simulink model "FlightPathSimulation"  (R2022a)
settings: Solver=VariableStepAuto  StartTime=0.0  StopTime=TF  RelTol=1e-3
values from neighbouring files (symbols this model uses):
  aircraft = RCAM_Transport    [RunSimulation.m]
undefined symbols (not defined in the file or in its folder): Column, Controls_0, D, deg, Earth, ft, km, m, rad, s, States_0, vector, WGS84
libraries: aerolibconvert2 x19, aerolibasang x3, aerolibadyn x1, aerolibatmos2 x1, shared6dof x1, aerolibtransform2 x1

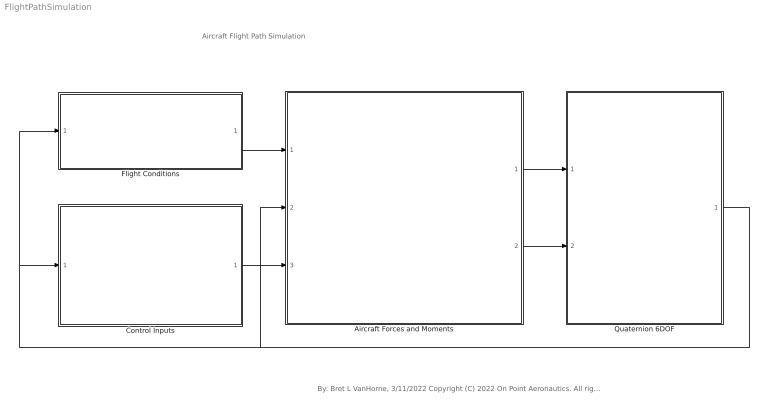
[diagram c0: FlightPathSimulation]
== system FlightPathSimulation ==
  note: Aircraft Flight Path Simulation
  note: By: Bret L VanHorne, 3/11/2022 Copyright (C) 2022 On Point Aeronautics. All rights reserved.
  Aircraft Forces and Moments : Subsystem
  Control Inputs : Subsystem
  Flight Conditions : Subsystem
  Quaternion 6DOF : Subsystem
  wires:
  Quaternion 6DOF/1(Bus Element Out13) -> Flight Conditions/1(Bus Element In2), Control Inputs/1(Bus Element In4), Aircraft Forces and Moments/3(States)
  Flight Conditions/1(Bus Element Out6) -> Aircraft Forces and Moments/1(Conditions)
  Control Inputs/1(Bus Element Out1) -> Aircraft Forces and Moments/2(Controls)
  Aircraft Forces and Moments/1(Forces) -> Quaternion 6DOF/1(Forces)
  Aircraft Forces and Moments/2(Moments) -> Quaternion 6DOF/2(Moments)

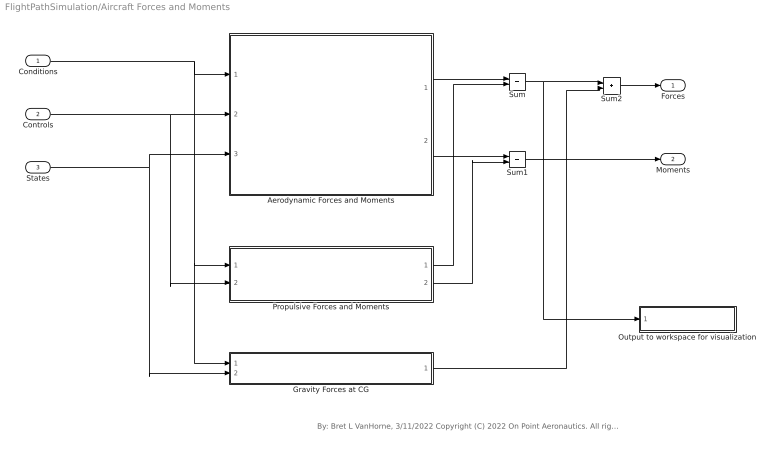
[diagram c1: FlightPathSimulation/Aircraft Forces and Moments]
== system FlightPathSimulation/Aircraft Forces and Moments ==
  note: By: Bret L VanHorne, 3/11/2022 Copyright (C) 2022 On Point Aeronautics. All rights reserved.
  Conditions : Inport
  Controls : Inport  Port=2
  States : Inport  Port=3
  Aerodynamic Forces and Moments : Subsystem
  Gravity Forces at CG : Subsystem
  Output to workspace for visualization : Subsystem
  Propulsive Forces and Moments : Subsystem
  Sum : Sum
  Sum1 : Sum
  Sum2 : Sum
  Forces : Outport
  Moments : Outport  Port=2
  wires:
  Aerodynamic Forces and Moments/1(Forces) -> Sum/1
  Propulsive Forces and Moments/1(Forces) -> Sum/2
  Aerodynamic Forces and Moments/2(Moments) -> Sum1/1
  Propulsive Forces and Moments/2(Moments) -> Sum1/2
  Conditions/1 -> Gravity Forces at CG/1(Bus Element In1), Propulsive Forces and Moments/1(Bus Element In), Aerodynamic Forces and Moments/1(Bus Element In9)
  Sum1/1 -> Moments/1
  Controls/1 -> Aerodynamic Forces and Moments/2(Bus Element In14), Propulsive Forces and Moments/2(Bus Element In2)
  States/1 -> Aerodynamic Forces and Moments/3(Bus Element In11), Gravity Forces at CG/2(Bus Element In2)
  Sum/1 -> Sum2/1, Output to workspace for visualization/1(In1)
  Gravity Forces at CG/1(Forces) -> Sum2/2
  Sum2/1 -> Forces/1

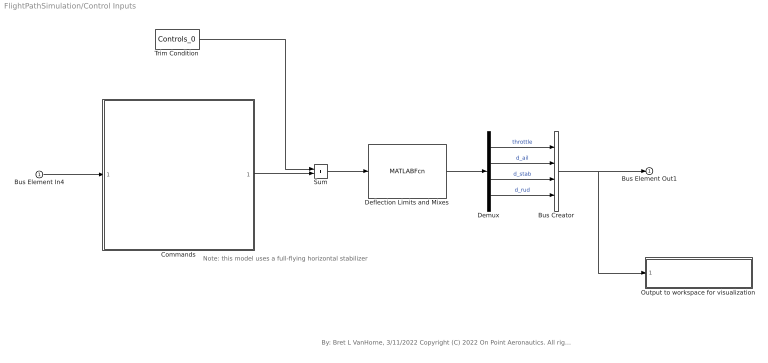
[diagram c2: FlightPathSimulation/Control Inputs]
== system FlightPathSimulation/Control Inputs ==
  note: Note: this model uses a full-flying horizontal stabilizer
  note: By: Bret L VanHorne, 3/11/2022 Copyright (C) 2022 On Point Aeronautics. All rights reserved.
  Bus Element In4 : Inport
  Bus Creator : BusCreator  Inputs=4
  Commands : Subsystem  ReferencedSubsystem=TurnCommands
  Deflection Limits and Mixes : MATLABFcn  MATLABFcn=aircraft.ControlRigging(u)
  Demux : Demux
  Output to workspace for visualization : Subsystem
  Sum : Sum
  Trim Condition : Constant  Value=Controls_0
  Bus Element Out1 : Outport
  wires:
  Sum/1 -> Deflection Limits and Mixes/1
  Trim Condition/1 -> Sum/1
  Bus Creator/1 -> Output to workspace for visualization/1(In1), Bus Element Out1/1
  Bus Element In4/1 -> Commands/1
  Commands/1 -> Sum/2
  Deflection Limits and Mixes/1 -> Demux/1
  Demux/1 -> Bus Creator/1  "throttle"
  Demux/2 -> Bus Creator/2  "d_ail"
  Demux/3 -> Bus Creator/3  "d_stab"
  Demux/4 -> Bus Creator/4  "d_rud"

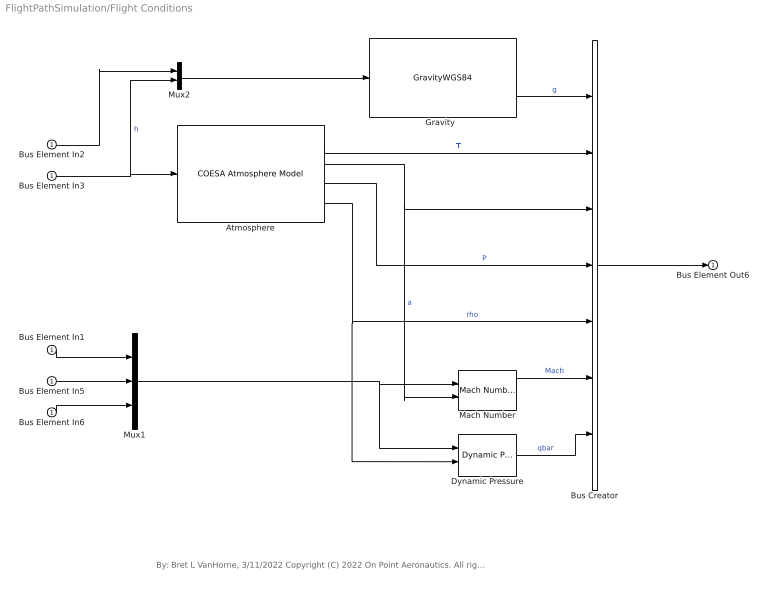
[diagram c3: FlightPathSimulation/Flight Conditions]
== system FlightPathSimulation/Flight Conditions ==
  note: By: Bret L VanHorne, 3/11/2022 Copyright (C) 2022 On Point Aeronautics. All rights reserved.
  Bus Element In{1..3,5..6} (5 alike) : Inport
  Atmosphere : aerolibatmos2/COESA Atmosphere Model  units=Metric (MKS)  spec=1976 COESA-extended U.S. Standard Atmosphere  model=Profile  profile_var=High temperature  profile_percent=1%  profile_alt=5 km (16404 ft)  envelope_var=High temperature  envelope_percent=1%  action=Warning
  Bus Creator : BusCreator  Inputs=7
  Dynamic Pressure : aerolibasang/Dynamic Pressure
  "Gravity  " : GravityWGS84
  Mach Number : aerolibasang/Mach Number
  Mux1 : Mux  Inputs=3
  Mux2 : Mux  Inputs=2
  Bus Element Out6 : Outport
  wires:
  Bus Element In6/1 -> Mux1/3
  Bus Element In5/1 -> Mux1/2
  Bus Element In2/1 -> Mux2/1
  Bus Element In1/1 -> Mux1/1
  Dynamic Pressure/1 -> Bus Creator/7  "qbar"
  Atmosphere/3 -> Bus Creator/4  "P"
  Atmosphere/1 -> Bus Creator/2  "T"
  Mux2/1 -> "Gravity  "/1
  Atmosphere/4 -> Dynamic Pressure/2, Bus Creator/5  "rho"
  "Gravity  "/1 -> Bus Creator/1  "g"
  Atmosphere/2 -> Mach Number/2, Bus Creator/3  "a"
  Mach Number/1 -> Bus Creator/6  "Mach"
  Bus Element In3/1 -> Mux2/2, Atmosphere/1  "h"
  Mux1/1 -> Dynamic Pressure/1, Mach Number/1
  Bus Creator/1 -> Bus Element Out6/1

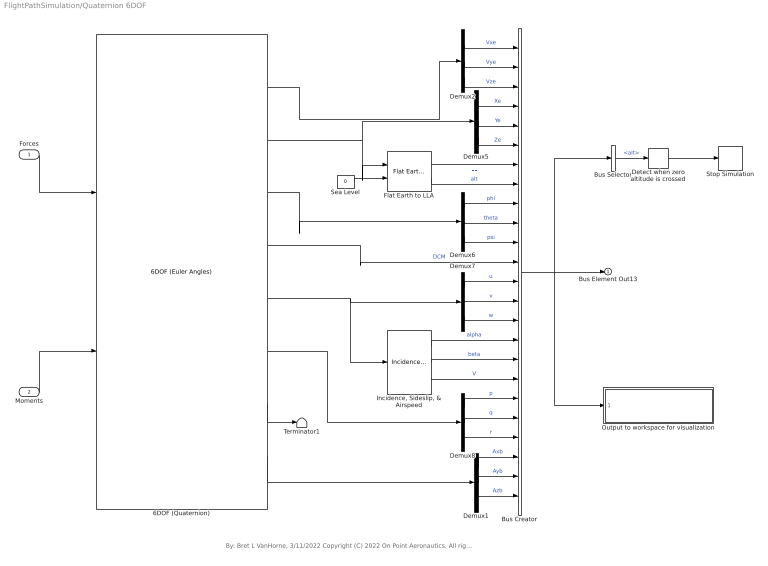
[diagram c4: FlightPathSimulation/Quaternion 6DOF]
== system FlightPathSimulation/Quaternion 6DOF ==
  note: By: Bret L VanHorne, 3/11/2022 Copyright (C) 2022 On Point Aeronautics. All rights reserved.
  Forces : Inport
  Moments : Inport  Port=2
  6DOF (Quaternion) : shared6dof/6DOF (Euler Angles)  units=Metric (MKS)  mtype=Fixed  rep=Quaternion  xme_0=States_0(1,:)  Vm_0=States_0(2,:)  eul_0=Euler_0  pm_0=States_0(3,:)  mass_0=aircraft.mass  mass_e=0.5  mass_f=2.0  inertia=aircraft.I  inertia_e=eye(3)  inertia_f=2*eye(3)  k_quat=1.0  vre_flag=on  abi_flag=off  aMode=0  xme_statename=''  Vm_statename=''  eul_statename=''  quat_statename=''  pm_statename=''  mass_statename=''
  Bus Selector : BusSelector  OutputSignals=alt
  Bus Creator : BusCreator  Inputs=24
  Demux{1..2,5..8} (6 alike) : Demux  Outputs=3
  Detect when zero altitude is crossed : HitCross
  Flat Earth to LLA : aerolibtransform2/Flat Earth to LLA  units=Metric (MKS)  ptype=Earth (WGS84)  F=1/298.257223563  R=6378137  refPosPort=off  LL0=[0 10]  psi=0
  "Incidence, Sideslip, & Airspeed" : aerolibasang/Incidence, Sideslip, & Airspeed
  Output to workspace for visualization : Subsystem
  Sea Level : Constant  Value=0
  Stop Simulation : Stop
  Terminator1 : Terminator
  Bus Element Out13 : Outport
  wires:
  Moments/1 -> 6DOF (Quaternion)/2
  Forces/1 -> 6DOF (Quaternion)/1
  6DOF (Quaternion)/2 -> Flat Earth to LLA/1, Demux5/1
  6DOF (Quaternion)/3 -> Demux6/1
  6DOF (Quaternion)/5 -> Demux7/1, "Incidence, Sideslip, & Airspeed"/1
  6DOF (Quaternion)/6 -> Demux8/1
  6DOF (Quaternion)/7 -> Terminator1/1
  6DOF (Quaternion)/1 -> Demux2/1
  Demux5/1 -> Bus Creator/4  "Xe"
  Demux5/2 -> Bus Creator/5  "Ye"
  Demux5/3 -> Bus Creator/6  "Ze"
  Demux6/1 -> Bus Creator/9  "phi"
  Demux6/2 -> Bus Creator/10  "theta"
  Demux6/3 -> Bus Creator/11  "psi"
  Demux7/1 -> Bus Creator/13  "u"
  Demux7/2 -> Bus Creator/14  "v"
  Demux7/3 -> Bus Creator/15  "w"
  Demux8/1 -> Bus Creator/19  "p"
  Demux8/2 -> Bus Creator/20  "q"
  Demux8/3 -> Bus Creator/21  "r"
  6DOF (Quaternion)/4 -> Bus Creator/12  "DCM"
  Bus Creator/1 -> Output to workspace for visualization/1(In1), Bus Element Out13/1, Bus Selector/1
  6DOF (Quaternion)/8 -> Demux1/1
  Demux1/1 -> Bus Creator/22  "Axb"
  Demux1/2 -> Bus Creator/23  "Ayb"
  Demux1/3 -> Bus Creator/24  "Azb"
  Bus Selector/1 -> Detect when zero altitude is crossed/1  "<alt>"
  Detect when zero altitude is crossed/1 -> Stop Simulation/1
  Demux2/1 -> Bus Creator/1  "Vxe"
  Demux2/2 -> Bus Creator/2  "Vye"
  Demux2/3 -> Bus Creator/3  "Vze"
  "Incidence, Sideslip, & Airspeed"/1 -> Bus Creator/16  "alpha"
  "Incidence, Sideslip, & Airspeed"/2 -> Bus Creator/17  "beta"
  "Incidence, Sideslip, & Airspeed"/3 -> Bus Creator/18  "V"
  Sea Level/1 -> Flat Earth to LLA/2
  Flat Earth to LLA/1 -> Bus Creator/7  "LL"
  Flat Earth to LLA/2 -> Bus Creator/8  "alt"

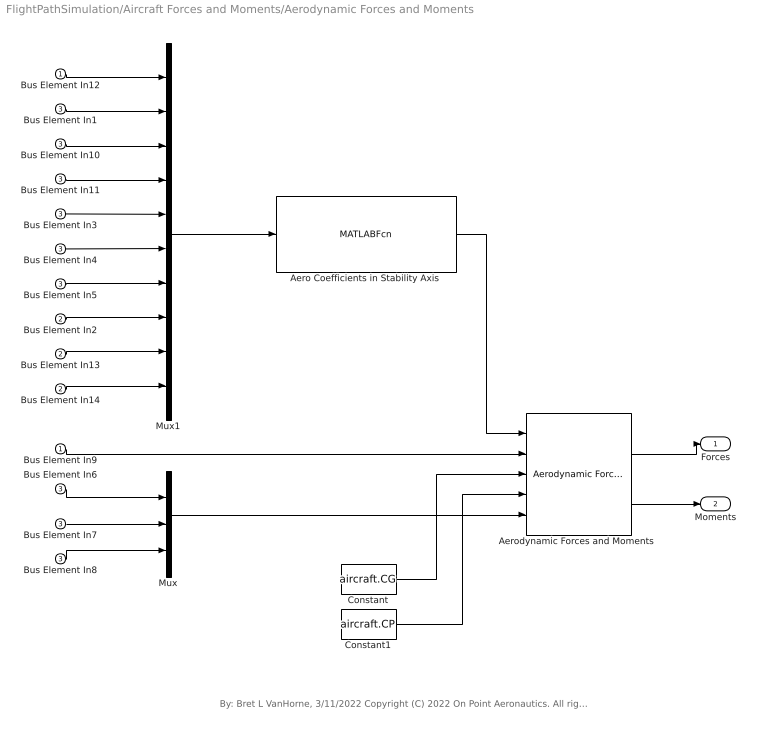
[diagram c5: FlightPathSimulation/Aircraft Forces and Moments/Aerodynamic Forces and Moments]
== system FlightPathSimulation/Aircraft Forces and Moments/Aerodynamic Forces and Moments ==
  note: By: Bret L VanHorne, 3/11/2022 Copyright (C) 2022 On Point Aeronautics. All rights reserved.
  Bus Element In9 : Inport
  Bus Element In12 : Inport
  Bus Element In2 : Inport  Port=2
  Bus Element In13 : Inport  Port=2
  Bus Element In14 : Inport  Port=2
  Bus Element In{1,3..8,10..11} (9 alike) : Inport  Port=3
  Aero Coefficients in Stability Axis : MATLABFcn  MATLABFcn=aircraft.AeroCoefficients(u(1), u(2:7), u(8:10))
  "Aerodynamic Forces and Moments " : aerolibadyn/Aerodynamic Forces and Moments   inputAxes=Stability  outputForceAxes=Body  outputMomentAxes=Body  S=aircraft.S  b=aircraft.b  cbar=aircraft.cbar
  Constant : Constant  Value=aircraft.CG
  Constant1 : Constant  Value=aircraft.CP
  Mux : Mux  Inputs=3
  Mux1 : Mux  Inputs=10
  Forces : Outport  Unit=N
  Moments : Outport  Port=2
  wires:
  Bus Element In9/1 -> "Aerodynamic Forces and Moments "/2
  Mux/1 -> "Aerodynamic Forces and Moments "/5
  Constant1/1 -> "Aerodynamic Forces and Moments "/4
  "Aerodynamic Forces and Moments "/2 -> Moments/1
  "Aerodynamic Forces and Moments "/1 -> Forces/1
  Constant/1 -> "Aerodynamic Forces and Moments "/3
  Bus Element In7/1 -> Mux/2
  Bus Element In8/1 -> Mux/3
  Bus Element In6/1 -> Mux/1
  Bus Element In1/1 -> Mux1/2
  Bus Element In14/1 -> Mux1/10
  Bus Element In10/1 -> Mux1/3
  Bus Element In11/1 -> Mux1/4
  Bus Element In12/1 -> Mux1/1
  Bus Element In3/1 -> Mux1/5
  Bus Element In4/1 -> Mux1/6
  Bus Element In5/1 -> Mux1/7
  Bus Element In2/1 -> Mux1/8
  Bus Element In13/1 -> Mux1/9
  Aero Coefficients in Stability Axis/1 -> "Aerodynamic Forces and Moments "/1
  Mux1/1 -> Aero Coefficients in Stability Axis/1

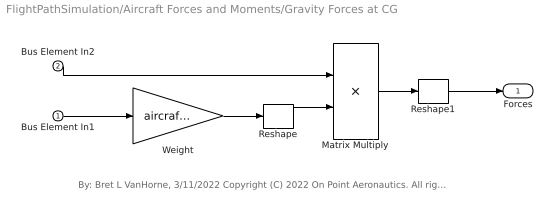
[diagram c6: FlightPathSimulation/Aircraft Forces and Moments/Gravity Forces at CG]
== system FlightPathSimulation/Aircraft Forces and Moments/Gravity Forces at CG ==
  note: By: Bret L VanHorne, 3/11/2022 Copyright (C) 2022 On Point Aeronautics. All rights reserved.
  Bus Element In1 : Inport
  Bus Element In2 : Inport  Port=2
  Matrix Multiply : Product  Multiplication=Matrix(*)
  Reshape : Reshape  OutputDimensionality=Column vector (2-D)
  Reshape1 : Reshape
  Weight : Gain  Gain=aircraft.mass
  Forces : Outport
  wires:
  Bus Element In1/1 -> Weight/1
  Weight/1 -> Reshape/1
  Bus Element In2/1 -> Matrix Multiply/1
  Reshape/1 -> Matrix Multiply/2
  Reshape1/1 -> Forces/1
  Matrix Multiply/1 -> Reshape1/1

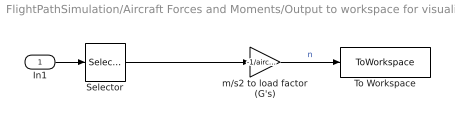
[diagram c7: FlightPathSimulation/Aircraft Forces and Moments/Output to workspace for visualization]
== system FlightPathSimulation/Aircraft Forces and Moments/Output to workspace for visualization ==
  In1 : Inport
  Selector : Selector  InputPortWidth=3  IndexOptions=Index vector (dialog)  Indices=[3]  OutputSizes=1
  To Workspace : ToWorkspace  VariableName=simAero  SaveFormat=Timeseries  SampleTime=-1
  m/s2 to load factor (G's) : Gain  Gain=-1/aircraft.weight
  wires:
  In1/1 -> Selector/1
  Selector/1 -> m/s2 to load factor (G's)/1
  m/s2 to load factor (G's)/1 -> To Workspace/1  "n"

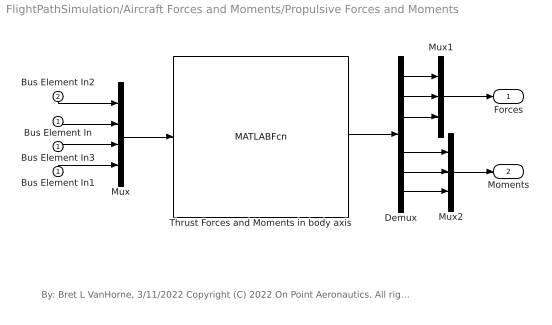
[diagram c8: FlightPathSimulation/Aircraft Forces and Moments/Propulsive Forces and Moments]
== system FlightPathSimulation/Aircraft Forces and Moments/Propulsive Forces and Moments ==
  note: By: Bret L VanHorne, 3/11/2022 Copyright (C) 2022 On Point Aeronautics. All rights reserved.
  Bus Element In : Inport
  Bus Element In1 : Inport
  Bus Element In3 : Inport
  Bus Element In2 : Inport  Port=2
  Demux : Demux  Outputs=6
  Mux : Mux
  Mux1 : Mux  Inputs=3
  Mux2 : Mux  Inputs=3
  Thrust Forces and Moments in body axis : MATLABFcn  MATLABFcn=aircraft.EngineThrust(u(1), u(2:4))
  Forces : Outport
  Moments : Outport  Port=2
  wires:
  Bus Element In2/1 -> Mux/1
  Bus Element In/1 -> Mux/2
  Bus Element In1/1 -> Mux/4
  Bus Element In3/1 -> Mux/3
  Mux/1 -> Thrust Forces and Moments in body axis/1
  Thrust Forces and Moments in body axis/1 -> Demux/1
  Mux1/1 -> Forces/1
  Demux/1 -> Mux1/1
  Demux/2 -> Mux1/2
  Demux/3 -> Mux1/3
  Demux/4 -> Mux2/1
  Demux/5 -> Mux2/2
  Demux/6 -> Mux2/3
  Mux2/1 -> Moments/1

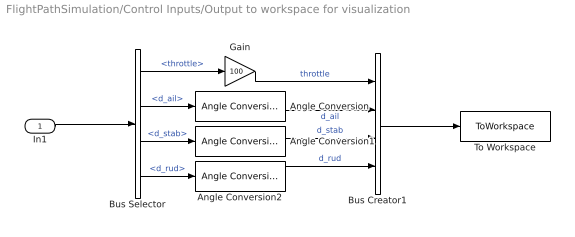
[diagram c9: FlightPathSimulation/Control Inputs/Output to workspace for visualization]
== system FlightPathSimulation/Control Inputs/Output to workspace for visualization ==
  In1 : Inport
  Angle Conversion : aerolibconvert2/Angle Conversion  IU=rad  OU=deg
  Angle Conversion1 : aerolibconvert2/Angle Conversion  IU=rad  OU=deg
  Angle Conversion2 : aerolibconvert2/Angle Conversion  IU=rad  OU=deg
  Bus Selector : BusSelector  OutputSignals=throttle,d_ail,d_stab,d_rud
  Bus Creator1 : BusCreator  Inputs=4
  Gain : Gain  Gain=100
  To Workspace : ToWorkspace  VariableName=simControls  SaveFormat=Timeseries  SampleTime=-1
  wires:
  Bus Selector/2 -> Angle Conversion/1  "<d_ail>"
  Bus Creator1/1 -> To Workspace/1
  Angle Conversion1/1 -> Bus Creator1/3  "d_stab"
  Bus Selector/1 -> Gain/1  "<throttle>"
  Angle Conversion2/1 -> Bus Creator1/4  "d_rud"
  Bus Selector/4 -> Angle Conversion2/1  "<d_rud>"
  Angle Conversion/1 -> Bus Creator1/2  "d_ail"
  Bus Selector/3 -> Angle Conversion1/1  "<d_stab>"
  In1/1 -> Bus Selector/1
  Gain/1 -> Bus Creator1/1  "throttle"

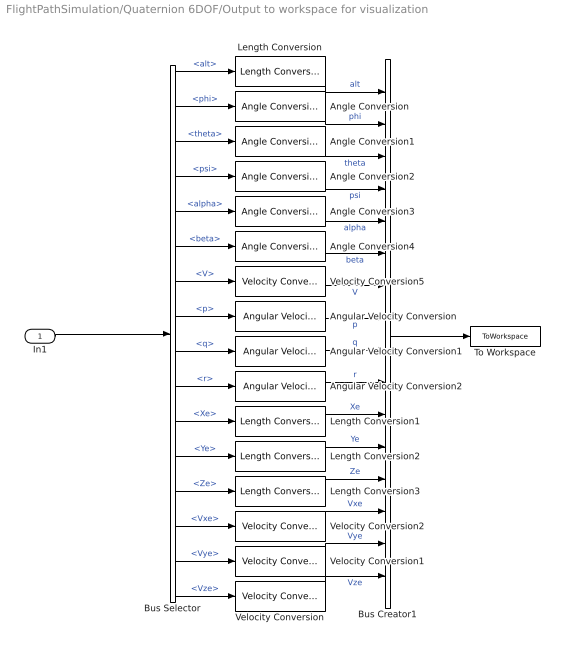
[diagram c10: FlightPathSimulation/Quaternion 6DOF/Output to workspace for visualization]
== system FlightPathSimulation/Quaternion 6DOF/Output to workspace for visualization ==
  In1 : Inport
  Angle Conversion{,1..4} (5 alike) : aerolibconvert2/Angle Conversion  IU=rad  OU=deg
  Angular Velocity Conversion : aerolibconvert2/Angular Velocity Conversion  IU=rad/s  OU=deg/s
  Angular Velocity Conversion1 : aerolibconvert2/Angular Velocity Conversion  IU=rad/s  OU=deg/s
  Angular Velocity Conversion2 : aerolibconvert2/Angular Velocity Conversion  IU=rad/s  OU=deg/s
  Bus Selector : BusSelector  OutputSignals=alt,phi,theta,psi,alpha,beta,V,p,q,r,Xe,Ye,Ze,Vxe,Vye,Vze
  Bus Creator1 : BusCreator  Inputs=16
  Length Conversion{,1..3} (4 alike) : aerolibconvert2/Length Conversion  IU=m  OU=ft
  To Workspace : ToWorkspace  VariableName=simStates  SaveFormat=Timeseries  SampleTime=-1
  Velocity Conversion{,1..2,5} (4 alike) : aerolibconvert2/Velocity Conversion  IU=m/s  OU=kts
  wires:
  Bus Selector/3 -> Angle Conversion1/1  "<theta>"
  Bus Selector/10 -> Angular Velocity Conversion2/1  "<r>"
  Bus Selector/9 -> Angular Velocity Conversion1/1  "<q>"
  Bus Selector/4 -> Angle Conversion2/1  "<psi>"
  Bus Creator1/1 -> To Workspace/1
  Angular Velocity Conversion/1 -> Bus Creator1/8  "p"
  Angle Conversion/1 -> Bus Creator1/2  "phi"
  Angular Velocity Conversion2/1 -> Bus Creator1/10  "r"
  Bus Selector/8 -> Angular Velocity Conversion/1  "<p>"
  Bus Selector/2 -> Angle Conversion/1  "<phi>"
  Angle Conversion1/1 -> Bus Creator1/3  "theta"
  In1/1 -> Bus Selector/1
  Angle Conversion2/1 -> Bus Creator1/4  "psi"
  Angular Velocity Conversion1/1 -> Bus Creator1/9  "q"
  Bus Selector/11 -> Length Conversion1/1  "<Xe>"
  Bus Selector/12 -> Length Conversion2/1  "<Ye>"
  Bus Selector/13 -> Length Conversion3/1  "<Ze>"
  Bus Selector/14 -> Velocity Conversion2/1  "<Vxe>"
  Bus Selector/15 -> Velocity Conversion1/1  "<Vye>"
  Bus Selector/16 -> Velocity Conversion/1  "<Vze>"
  Velocity Conversion1/1 -> Bus Creator1/15  "Vye"
  Velocity Conversion2/1 -> Bus Creator1/14  "Vxe"
  Velocity Conversion/1 -> Bus Creator1/16  "Vze"
  Bus Selector/5 -> Angle Conversion3/1  "<alpha>"
  Angle Conversion3/1 -> Bus Creator1/5  "alpha"
  Bus Selector/6 -> Angle Conversion4/1  "<beta>"
  Bus Selector/7 -> Velocity Conversion5/1  "<V>"
  Velocity Conversion5/1 -> Bus Creator1/7  "V"
  Angle Conversion4/1 -> Bus Creator1/6  "beta"
  Bus Selector/1 -> Length Conversion/1  "<alt>"
  Length Conversion/1 -> Bus Creator1/1  "alt"
  Length Conversion3/1 -> Bus Creator1/13  "Ze"
  Length Conversion2/1 -> Bus Creator1/12  "Ye"
  Length Conversion1/1 -> Bus Creator1/11  "Xe"
